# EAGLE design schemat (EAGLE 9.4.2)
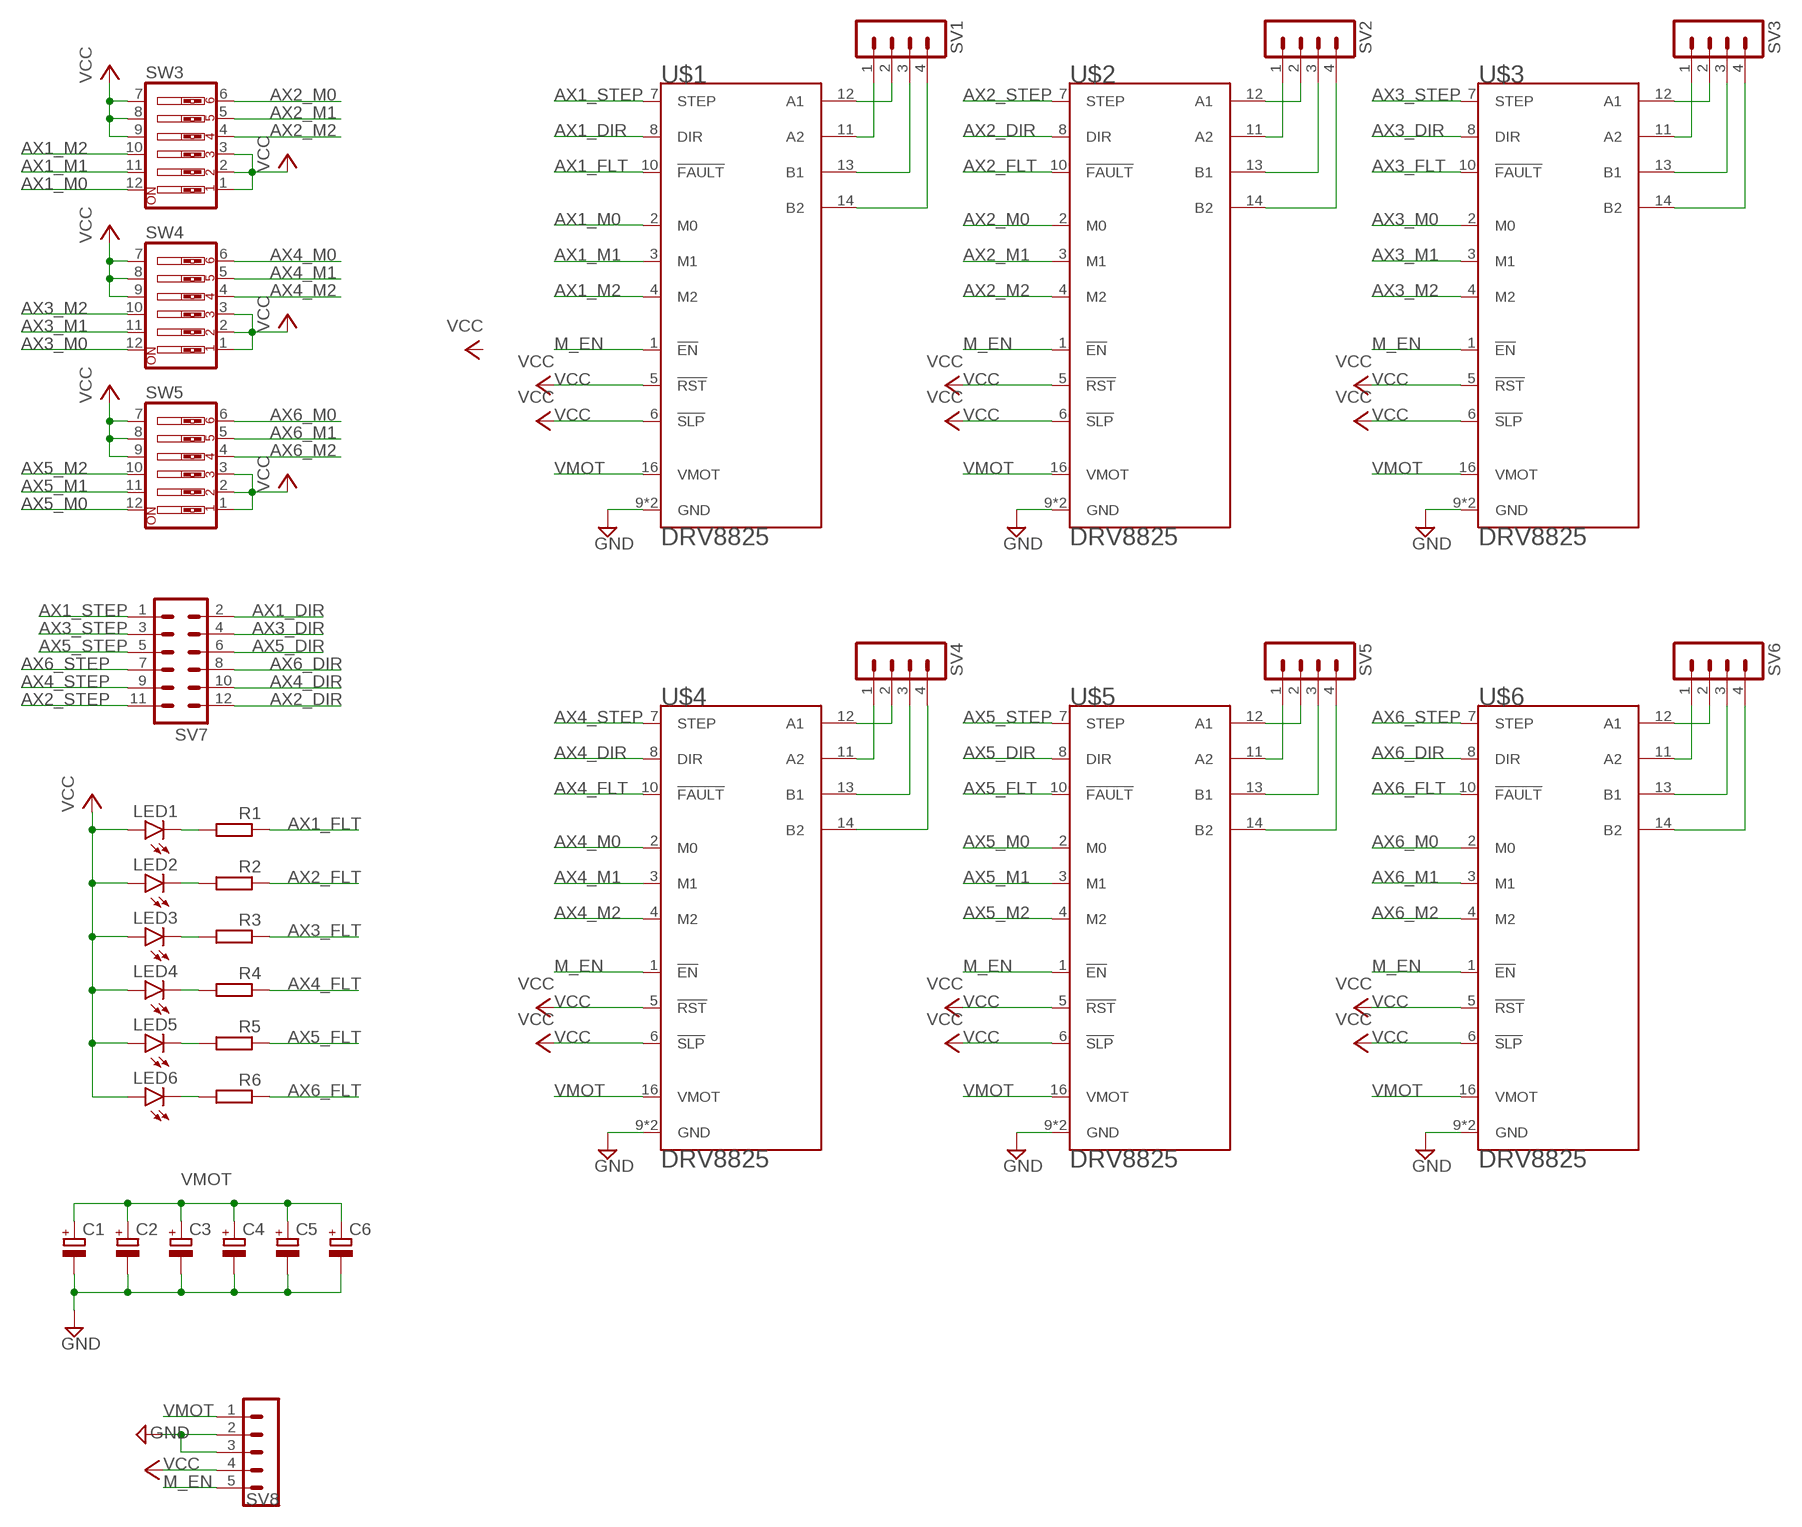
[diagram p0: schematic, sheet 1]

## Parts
C1  CPOL-EUE2.5-7  [E2,5-7]
C2  CPOL-EUE2.5-7  [E2,5-7]
C3  CPOL-EUE2.5-7  [E2,5-7]
C4  CPOL-EUE2.5-7  [E2,5-7]
C5  CPOL-EUE2.5-7  [E2,5-7]
C6  CPOL-EUE2.5-7  [E2,5-7]
LED1  LED5MM  [LED5MM]
LED2  LED5MM  [LED5MM]
LED3  LED5MM  [LED5MM]
LED4  LED5MM  [LED5MM]
LED5  LED5MM  [LED5MM]
LED6  LED5MM  [LED5MM]
R1  R-EU_0207/10  [0207/10]
R2  R-EU_0207/10  [0207/10]
R3  R-EU_0207/10  [0207/10]
R4  R-EU_0207/10  [0207/10]
R5  R-EU_0207/10  [0207/10]
R6  R-EU_0207/10  [0207/10]
SV1  MA04-1  [MA04-1]
SV2  MA04-1  [MA04-1]
SV3  MA04-1  [MA04-1]
SV4  MA04-1  [MA04-1]
SV5  MA04-1  [MA04-1]
SV6  MA04-1  [MA04-1]
SV7  MA06-2  [MA06-2]
SV8  MA05-1  [MA05-1]
SW3  SW_DIP-6  [EDG-06]
SW4  SW_DIP-6  [EDG-06]
SW5  SW_DIP-6  [EDG-06]
U$1  DRV8825  [DRV8825]
U$2  DRV8825  [DRV8825]
U$3  DRV8825  [DRV8825]
U$4  DRV8825  [DRV8825]
U$5  DRV8825  [DRV8825]
U$6  DRV8825  [DRV8825]

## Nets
AX1_DIR: SV7.2 U$1.8(DIR)
AX1_FLT: R1.1 U$1.10(!FAULT)
AX1_M0: SW3.12 U$1.2(M0)
AX1_M1: SW3.11 U$1.3(M1)
AX1_M2: SW3.10 U$1.4(M2)
AX1_STEP: SV7.1 U$1.7(STEP)
AX2_DIR: SV7.12 U$2.8(DIR)
AX2_FLT: R2.1 U$2.10(!FAULT)
AX2_M0: SW3.6 U$2.2(M0)
AX2_M1: SW3.5 U$2.3(M1)
AX2_M2: SW3.4 U$2.4(M2)
AX2_STEP: SV7.11 U$2.7(STEP)
AX3_DIR: SV7.4 U$3.8(DIR)
AX3_FLT: R3.1 U$3.10(!FAULT)
AX3_M0: SW4.12 U$3.2(M0)
AX3_M1: SW4.11 U$3.3(M1)
AX3_M2: SW4.10 U$3.4(M2)
AX3_STEP: SV7.3 U$3.7(STEP)
AX4_DIR: SV7.10 U$4.8(DIR)
AX4_FLT: R4.1 U$4.10(!FAULT)
AX4_M0: SW4.6 U$4.2(M0)
AX4_M1: SW4.5 U$4.3(M1)
AX4_M2: SW4.4 U$4.4(M2)
AX4_STEP: SV7.9 U$4.7(STEP)
AX5_DIR: SV7.6 U$5.8(DIR)
AX5_FLT: R5.1 U$5.10(!FAULT)
AX5_M0: SW5.12 U$5.2(M0)
AX5_M1: SW5.11 U$5.3(M1)
AX5_M2: SW5.10 U$5.4(M2)
AX5_STEP: SV7.5 U$5.7(STEP)
AX6_DIR: SV7.8 U$6.8(DIR)
AX6_FLT: R6.1 U$6.10(!FAULT)
AX6_M0: SW5.6 U$6.2(M0)
AX6_M1: SW5.5 U$6.3(M1)
AX6_M2: SW5.4 U$6.4(M2)
AX6_STEP: SV7.7 U$6.7(STEP)
GND: C1.- C2.- C3.- C4.- C5.- C6.- SV8.2 SV8.3 U$1.9(GND) U$1.15(GND) U$2.9(GND) U$2.15(GND) U$3.9(GND) U$3.15(GND) U$4.9(GND) U$4.15(GND) U$5.9(GND) U$5.15(GND) U$6.9(GND) U$6.15(GND)
M_EN: SV8.5 U$1.1(!EN) U$2.1(!EN) U$3.1(!EN) U$4.1(!EN) U$5.1(!EN) U$6.1(!EN)
N$1: SV4.1 U$4.11(A2)
N$2: LED1.K(C) R1.2
N$3: LED2.K(C) R2.2
N$4: LED3.K(C) R3.2
N$5: LED4.K(C) R4.2
N$6: LED5.K(C) R5.2
N$7: SV4.2 U$4.12(A1)
N$8: LED6.K(C) R6.2
N$9: SV5.2 U$5.12(A1)
N$10: SV5.1 U$5.11(A2)
N$11: SV6.2 U$6.12(A1)
N$12: SV6.1 U$6.11(A2)
N$13: SV3.2 U$3.12(A1)
N$14: SV3.1 U$3.11(A2)
N$15: SV2.2 U$2.12(A1)
N$16: SV2.1 U$2.11(A2)
N$17: SV1.2 U$1.12(A1)
N$18: SV1.1 U$1.11(A2)
N$21: SV1.4 U$1.14(B2)
N$22: SV1.3 U$1.13(B1)
N$25: SV2.4 U$2.14(B2)
N$26: SV2.3 U$2.13(B1)
N$29: SV5.4 U$5.14(B2)
N$30: SV5.3 U$5.13(B1)
N$33: SV6.4 U$6.14(B2)
N$34: SV6.3 U$6.13(B1)
N$35: SV4.3 U$4.13(B1)
N$36: SV4.4 U$4.14(B2)
N$41: SV3.4 U$3.14(B2)
N$42: SV3.3 U$3.13(B1)
VCC: LED1.A LED2.A LED3.A LED4.A LED5.A LED6.A SV8.4 SW3.1 SW3.2 SW3.3 SW3.7 SW3.8 SW3.9 SW4.1 SW4.2 SW4.3 SW4.7 SW4.8 SW4.9 SW5.1 SW5.2 SW5.3 SW5.7 SW5.8 SW5.9 U$1.5(!RST) U$1.6(!SLP) U$2.5(!RST) U$2.6(!SLP) U$3.5(!RST) U$3.6(!SLP) U$4.5(!RST) U$4.6(!SLP) U$5.5(!RST) U$5.6(!SLP) U$6.5(!RST) U$6.6(!SLP)
VMOT: C1.+ C2.+ C3.+ C4.+ C5.+ C6.+ SV8.1 U$1.16(VMOT) U$2.16(VMOT) U$3.16(VMOT) U$4.16(VMOT) U$5.16(VMOT) U$6.16(VMOT)

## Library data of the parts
C1-C6 = my-rcl:CPOL-EU: POLARIZED CAPACITOR, European symbol; SPICEPREFIX: C
LED1-LED6 = myled:LED: LED
R1-R6 = rcl2:R-EU_: RESISTOR, European symbol; SPICEPREFIX: R
SV1-SV6 = con-lstb:MA04-1: PIN HEADER; OC_FARNELL: unknown; OC_NEWARK: unknown
SV7 = my-con-lstb:MA06-2: PIN HEADER; OC_FARNELL: unknown; OC_NEWARK: unknown
SV8 = con-lstb:MA05-1: PIN HEADER; OC_FARNELL: unknown; OC_NEWARK: unknown
SW3-SW5 = special:SW_DIP-6: DIP SWITCH
U$1-U$6 = robot-driver:DRV8825

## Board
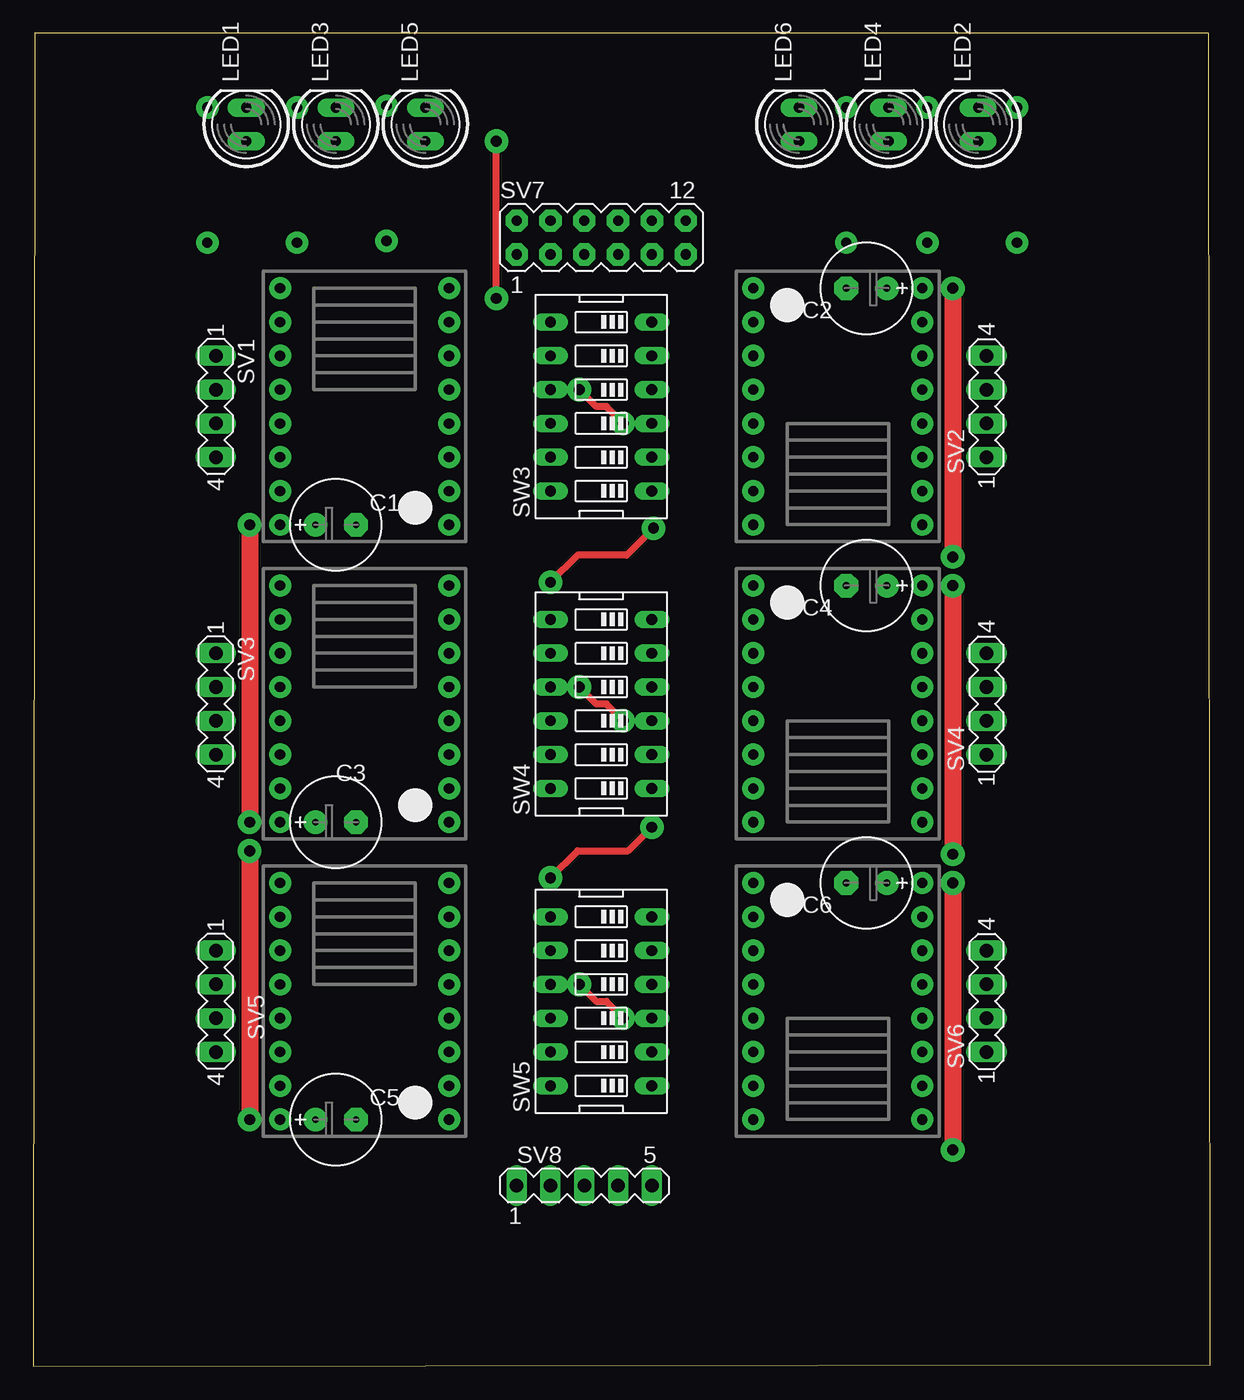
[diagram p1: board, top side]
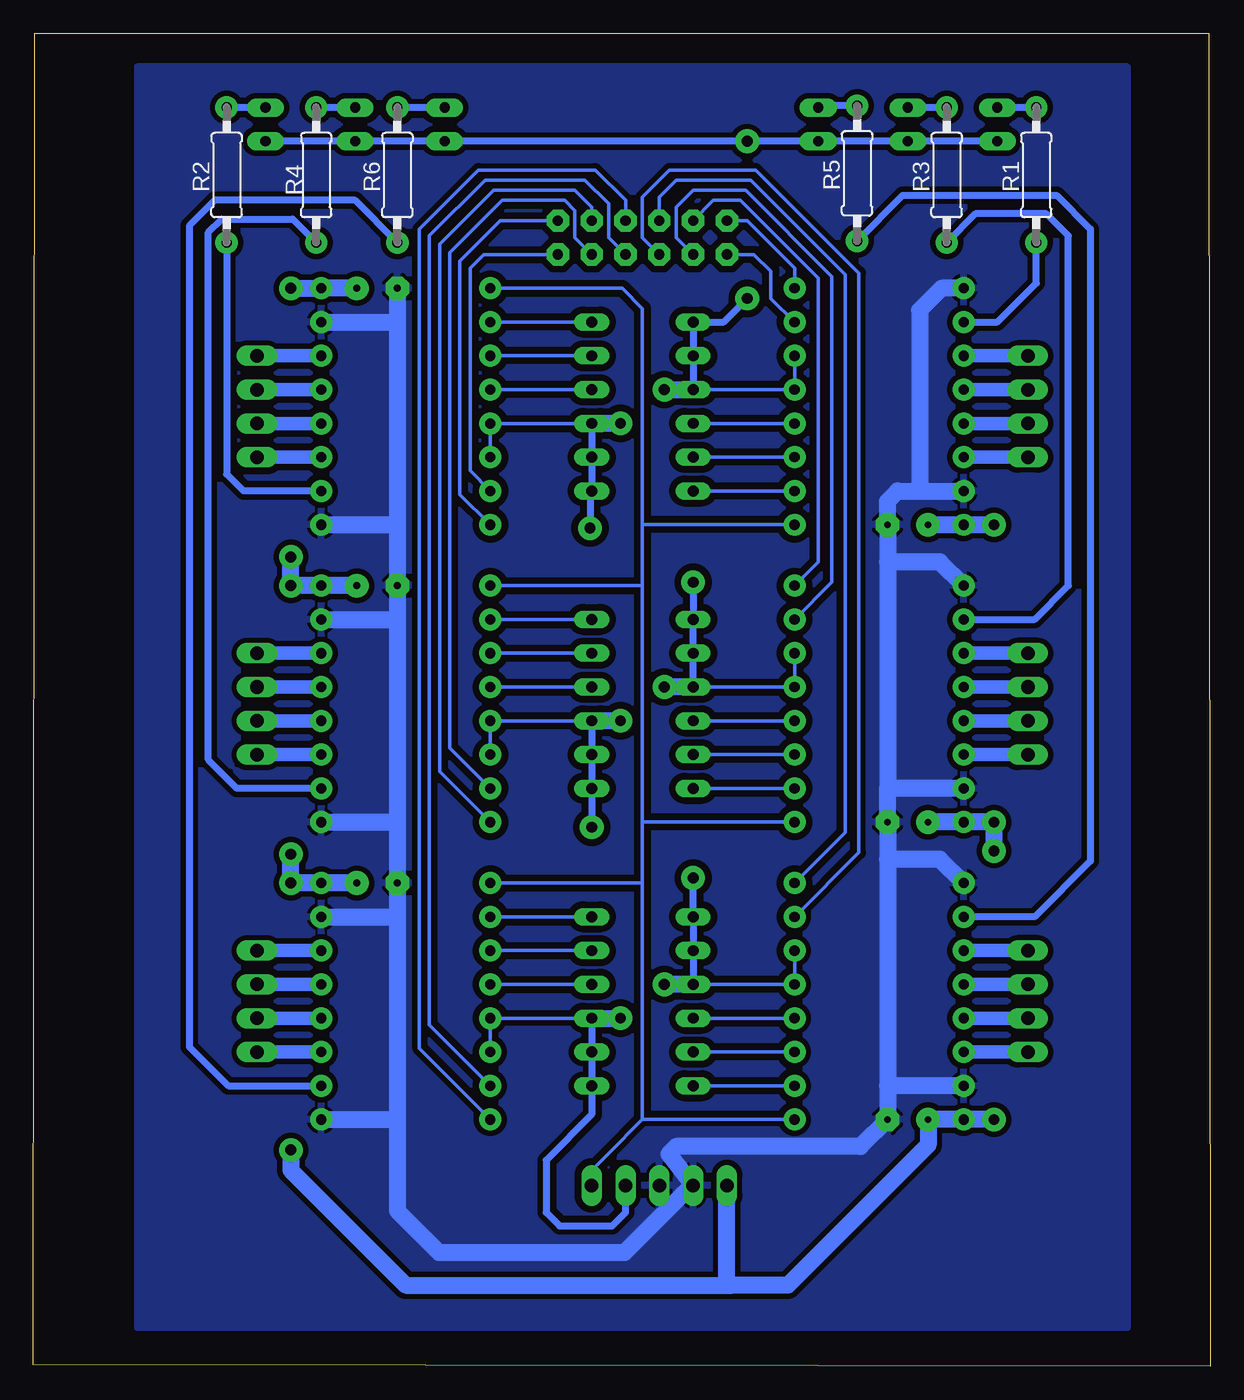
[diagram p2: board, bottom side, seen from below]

Size 88.44 x 100.19 mm. Coordinates in mm from the lower left corner, seen from the top.
Outline: 0,0 88.44,0.13 88.32,100.19 0.13,100.19 0,0
Copper layers (1*16): Top 0.035mm / dielectric 1.5mm / Bottom 0.035mm
Design rules "default *": minimum track width 6mil, minimum drill 0.35mm, track to track 8mil, track to pad 8mil, pad to pad 10mil, via to via 10mil, smd to smd 6mil, copper to edge 40mil, drill to drill 6mil, minimum pad ring 10mil, minimum via ring 8mil, stop-mask expansion 4mil, vias tented up to drill 0mil, thermal gap 10mil

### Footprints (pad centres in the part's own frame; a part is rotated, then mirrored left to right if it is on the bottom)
E2,5-7 = drill 0.508 pad 1.778: + -1.524,0 | drill 0.508 pad 1.778 octagon: - 1.524,0
LED5MM = drill 0.762 pad 1.397 long: A -1.27,0; K 1.27,0
0207/10 = drill 0.762 pad 1.676: 1 -5.08,0; 2 5.08,0
MA04-1 = drill 1.016 long: 1 -3.81,0; 2 -1.27,0; 3 1.27,0; 4 3.81,0
MA06-2 = drill 0.762 pad 1.676 octagon: 1 -6.35,-1.27; 2 -6.35,1.27; 3 -3.81,-1.27; 4 -3.81,1.27; 5 -1.27,-1.27; 6 -1.27,1.27; 7 1.27,-1.27; 8 1.27,1.27; 9 3.81,-1.27; 10 3.81,1.27; 11 6.35,-1.27; 12 6.35,1.27
MA05-1 = drill 1.016 long: 1 -5.08,0; 2 -2.54,0; 3 0,0; 4 2.54,0; 5 5.08,0
EDG-06 = drill 0.813 long: 1 -6.35,-3.81; 2 -3.81,-3.81; 3 -1.27,-3.81; 4 1.27,-3.81; 5 3.81,-3.81; 6 6.35,-3.81; 7 6.35,3.81; 8 3.81,3.81; 9 1.27,3.81; 10 -1.27,3.81; 11 -3.81,3.81; 12 -6.35,3.81
DRV8825 = drill 0.762 pad 1.651: 1 -6.35,8.89; 2 -6.35,6.35; 3 -6.35,3.81; 4 -6.35,1.27; 5 -6.35,-1.27; 6 -6.35,-3.81; 7 -6.35,-6.35; 8 -6.35,-8.89; 9 6.35,-8.89; 10 6.35,-6.35; 11 6.35,-3.81; 12 6.35,-1.27; 13 6.35,1.27; 14 6.35,3.81; 15 6.35,6.35; 16 6.35,8.89

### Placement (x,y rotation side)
C1  22.73,63.25 0 top
C2  62.61,81.03 180 top
C3  22.73,40.89 0 top
C4  62.61,58.67 180 top
C5  22.73,18.54 0 top
C6  62.61,36.32 180 top
LED1  16,93.34 90 top
LED2  70.99,93.34 90 top
LED3  22.73,93.34 90 top
LED4  64.26,93.34 90 top
LED5  29.46,93.34 90 top
LED6  57.53,93.34 90 top
R1  13.08,89.53 90 bottom
R2  73.91,89.53 90 bottom
R3  19.81,89.53 90 bottom
R4  67.18,89.53 90 bottom
R5  26.54,89.66 90 bottom
R6  61.09,89.53 90 bottom
SV1  13.72,72.14 270 top
SV2  71.63,72.14 90 top
SV3  13.72,49.78 270 top
SV4  71.63,49.78 90 top
SV5  13.72,27.43 270 top
SV6  71.63,27.43 90 top
SV7  42.67,84.84 0 top
SV8  41.4,13.59 0 top
SW3  42.67,72.14 90 top
SW4  42.67,49.78 90 top
SW5  42.67,27.43 90 top
U$1  24.89,72.14 180 top
U$2  60.45,72.14 0 top
U$3  24.89,49.78 180 top
U$4  60.45,49.78 0 top
U$5  24.89,27.43 180 top
U$6  60.45,27.43 0 top

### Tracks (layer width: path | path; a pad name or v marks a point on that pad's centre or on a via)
AX1_DIR
  Bottom 0.254: U$1.8 31.24,82.55 34.8,86.11 SV7.2
AX1_FLT
  Bottom 0.508: U$1.10 16,78.49 13.08,81.41 R1.1
AX1_M0
  Bottom 0.254: U$1.2 SW3.12
AX1_M1
  Bottom 0.254: U$1.3 SW3.11
AX1_M2
  Bottom 0.254: U$1.4 SW3.10
AX1_STEP
  Bottom 0.254: U$1.7 33.02,80.26 33.02,82.3 34.29,83.57 SV7.1
AX2_DIR
  Bottom 0.254: U$2.8 56.39,65.53 56.39,83.06 53.34,86.11 SV7.12
AX2_FLT
  Bottom 0.508: U$2.10 72.64,65.79 73.91,67.06 R2.1
AX2_M0
  Bottom 0.254: SW3.6 U$2.2
AX2_M1
  Bottom 0.254: SW3.5 U$2.3
AX2_M2
  Bottom 0.254: SW3.4 U$2.4
AX2_STEP
  Bottom 0.254: U$2.7 55.63,67.31 55.63,82.55 54.61,83.57 SV7.11
AX3_DIR
  Bottom 0.254: U$3.8 29.46,60.45 29.46,81.79 35.31,87.63 37.34,87.63 SV7.4
AX3_FLT
  Bottom 0.508: U$3.10 13.21,56.13 10.67,58.67 10.67,84.96 12.32,86.61 17.65,86.61 R3.1
AX3_M0
  Bottom 0.254: U$3.2 SW4.12
AX3_M1
  Bottom 0.254: U$3.3 SW4.11
AX3_M2
  Bottom 0.254: U$3.4 SW4.10
AX3_STEP
  Bottom 0.254: U$3.7 28.45,58.93 28.45,81.92 34.92,88.39 38.86,88.39 40.13,87.12 40.13,84.84 SV7.3
AX4_DIR
  Bottom 0.254: U$4.8 57.91,44.7 57.91,84.33 53.85,88.39 47.75,88.39 46.48,87.12 SV7.10
AX4_FLT
  Bottom 0.508: U$4.10 73.15,43.43 75.29,45.57 75.29,85.24 74.3,86.23 68.96,86.23 R4.1
AX4_M0
  Bottom 0.254: U$4.2 SW4.6
AX4_M1
  Bottom 0.254: U$4.3 SW4.5
AX4_M2
  Bottom 0.254: U$4.4 SW4.4
AX4_STEP
  Bottom 0.254: U$4.7 57.15,46.48 57.15,83.69 53.21,87.63 48.51,87.63 47.75,86.87 47.75,84.84 SV7.9
AX5_DIR
  Bottom 0.254: U$5.8 27.43,40.13 27.43,82.04 34.54,89.15 40.13,89.15 41.4,87.88 SV7.6
AX5_FLT
  Bottom 0.508: R5.1 23.11,88.01 11.56,88.01 9.02,85.47 9.02,37.97 13.21,33.78 U$5.10
AX5_M0
  Bottom 0.254: U$5.2 SW5.12
AX5_M1
  Bottom 0.254: U$5.3 SW5.11
AX5_M2
  Bottom 0.254: U$5.4 SW5.10
AX5_STEP
  Bottom 0.254: U$5.7 26.42,38.61 26.42,82.17 34.16,89.92 40.64,89.92 42.67,87.88 42.67,84.84 SV7.5
AX6_DIR
  Bottom 0.254: U$6.8 59.44,23.88 59.44,85.47 54.99,89.92 46.23,89.92 43.94,87.63 SV7.8
AX6_FLT
  Bottom 0.508: R6.1 64.26,87.63 74.8,87.63 76.71,85.73 76.71,24 73.79,21.08 U$6.10
AX6_M0
  Bottom 0.254: U$6.2 SW5.6
AX6_M1
  Bottom 0.254: U$6.3 SW5.5
AX6_M2
  Bottom 0.254: U$6.4 SW5.4
AX6_STEP
  Bottom 0.254: U$6.7 58.67,25.65 58.67,84.96 54.48,89.15 46.99,89.15 45.21,87.38 45.21,84.84 SV7.7
GND
  Bottom 1.27: 21.84,65.79 23.49,65.79 24.26,65.02 C1.- 24.26,60.45 | 21.84,65.79 U$1.15 | U$6.15 61.21,33.78 61.09,33.91 | 24.26,60.45 24.26,43.43 | 24.26,38.1 C3.- 24.26,43.43 | 24.26,38.1 24.26,21.08 | 24.26,21.08 C5.- 26.29,16.51 40.13,16.51 40.68,15.96 SV8.2 39.13,13.45 44.02,8.56 57.96,8.56 61.09,11.68 61.09,18.54 | C2.- 61.09,78.49 | 61.09,78.49 61.09,63.25 | 61.09,63.25 C4.- 61.09,56.01 | 61.09,56.01 61.09,40.89 | 61.09,40.89 C6.- 61.09,33.91 | 61.09,33.91 61.09,18.54 | U$5.9 20.32,38.1 24.26,38.1 | U$3.9 20.32,60.45 24.26,60.45 | U$1.9 20.19,81.03 21.84,79.38 21.84,65.79 | U$2.9 61.09,63.25 | U$4.9 61.09,40.89 | U$6.9 61.09,18.54 | U$2.15 61.09,78.49 | U$4.15 61.21,56.13 61.09,56.01 | U$3.15 24.26,43.43 | U$5.15 24.26,21.08
  pour Bottom (isolate 0.406): 6.22,97.66 80.64,97.66 80.64,2.92 6.22,2.92
M_EN
  Bottom 0.254: 42.67,63.25 42.67,79.5 44.2,81.03 U$2.1 | 42.67,63.25 42.67,58.67 | 42.67,58.67 42.67,40.89 | 42.67,40.89 42.67,36.32 | U$1.1 42.67,63.25 | U$4.1 42.67,58.67 | U$6.1 42.67,36.32 | U$3.1 42.67,40.89 | U$5.1 42.67,18.54 | 42.67,36.32 42.67,18.54 | 42.67,18.54 45.28,15.94 46.48,14.73 SV8.5
N$1
  Bottom 1.016: U$4.11 SV4.1
N$2
  Bottom 0.508: R1.2 LED1.K
N$3
  Bottom 0.508: LED2.K R2.2
N$4
  Bottom 0.508: R3.2 LED3.K
N$5
  Bottom 0.508: LED4.K R4.2
N$6
  Bottom 0.508: R5.2 29.34,94.74 LED5.K
N$7
  Bottom 1.016: U$4.12 SV4.2
N$8
  Bottom 0.508: LED6.K R6.2
N$9
  Bottom 1.016: SV5.2 U$5.12
N$10
  Bottom 1.016: SV5.1 U$5.11
N$11
  Bottom 1.016: U$6.12 SV6.2
N$12
  Bottom 1.016: U$6.11 SV6.1
N$13
  Bottom 1.016: SV3.2 U$3.12
N$14
  Bottom 1.016: SV3.1 U$3.11
N$15
  Bottom 1.016: U$2.12 SV2.2
N$16
  Bottom 1.016: U$2.11 SV2.1
N$17
  Bottom 1.016: SV1.2 U$1.12
N$18
  Bottom 1.016: SV1.1 U$1.11
N$19
  pour Bottom (isolate 0.508): 8.76,97.28 77.6,97.28 77.6,9.65 8.76,9.65
N$21
  Bottom 1.016: SV1.4 U$1.14
N$22
  Bottom 1.016: SV1.3 U$1.13
N$25
  Bottom 1.016: U$2.14 SV2.4
N$26
  Bottom 1.016: U$2.13 SV2.3
N$29
  Bottom 1.016: SV5.4 U$5.14
N$30
  Bottom 1.016: SV5.3 U$5.13
N$33
  Bottom 1.016: U$6.14 SV6.4
N$34
  Bottom 1.016: U$6.13 SV6.3
N$35
  Bottom 1.016: U$4.13 SV4.3
N$36
  Bottom 1.016: U$4.14 SV4.4
N$41
  Bottom 1.016: SV3.4 U$3.14
N$42
  Bottom 1.016: SV3.3 U$3.13
VCC  (via drill 0.81 pad 1.78)
  Top 0.508: v46.61,62.99 44.58,60.96 40.89,60.96 v38.86,58.93 | v44.32,70.87 43.05,72.14 42.29,72.14 v41.02,73.41 | v44.32,48.51 43.05,49.78 42.29,49.78 v41.02,51.05 | v38.86,36.7 40.89,38.73 44.7,38.73 v46.48,40.51 | v41.02,28.7 42.29,27.43 43.05,27.43 v44.32,26.16 | v34.8,80.26 v34.8,92.08
  Bottom 0.254: U$6.6 U$6.5 SW5.3 | U$5.6 U$5.5 SW5.9 | U$3.6 U$3.5 SW4.9 | U$4.6 54.1,48.39 | 54.1,48.39 U$4.5 | SW4.3 53.97,48.51 54.1,48.39 | U$1.6 U$1.5 SW3.9 | U$2.6 U$2.5 SW3.3
  Bottom 0.508: SW4.3 SW4.2 SW4.1 v46.48,40.51 | SW4.9 SW4.8 SW4.7 v38.86,58.93 | SW3.3 SW3.2 SW3.1 46.61,65.66 v46.61,62.99 | SW3.9 SW3.8 SW3.7 36.58,78.49 v34.8,80.26 | SW5.9 SW5.8 SW5.7 v38.86,36.7 | SW5.3 SW5.2 SW5.1 46.48,18.92 49.91,15.49 49.91,11.56 48.89,10.54 44.96,10.54 43.94,11.56 SV8.4 | LED1.A LED3.A LED5.A v34.8,92.08 LED6.A LED4.A LED2.A
  Bottom 1.27: SW4.9 v41.02,51.05 | v44.32,48.51 SW4.3 | SW5.9 v41.02,28.7 | SW5.3 v44.32,26.16 | v44.32,70.87 SW3.3 | v41.02,73.41 SW3.9
VMOT  (via drill 0.81 pad 1.78)
  Top 1.27: v16.26,63.25 v16.26,40.89 | v16.26,38.73 v16.26,18.54 | v69.09,81.03 v69.09,60.83 | v69.09,58.67 v69.09,38.48 | v69.09,36.32 v69.09,16.26
  Bottom 1.27: C1.+ U$1.16 v16.26,63.25 | C3.+ U$3.16 v16.26,40.89 v16.26,38.73 | C2.+ U$2.16 v69.09,81.03 | C4.+ U$4.16 v69.09,58.67 v69.09,60.83 | C6.+ U$6.16 v69.09,36.32 v69.09,38.48 | v16.26,18.54 U$5.16 C5.+ 21.21,16.64 31.75,6.1 35.94,6.1 | SV8.1 36.32,6.16 35.94,6.1 | v69.09,16.26 69.09,14.73 60.45,6.1 35.94,6.1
